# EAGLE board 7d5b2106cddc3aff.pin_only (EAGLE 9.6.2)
REV: A

Size 17.78 x 12.7 mm. Coordinates in mm from the lower left corner, seen from the top.
Outline: 0,10.16 0,2.54 arc90 2.54,0 15.24,0 arc90 17.78,2.54 17.78,10.16 arc90 15.24,12.7 2.54,12.7 arc90 0,10.16
Copper layers (1*16): Top 0.035mm / dielectric 1.5mm / Bottom 0.035mm
Design rules "adafruit *": minimum track width 8mil, minimum drill 15.5mil, track to track 8mil, track to pad 8mil, pad to pad 8mil, via to via 8mil, smd to smd 8mil, copper to edge 10mil, drill to drill 8mil, minimum pad ring 10mil, minimum via ring 8mil, stop-mask expansion 2mil, vias tented up to drill 20mil, thermal gap 10mil
Net classes: 1 highpower: width 0.305 mm, drill 0.483 mm; 2 lowpower: width 0.254 mm, drill 0.483 mm

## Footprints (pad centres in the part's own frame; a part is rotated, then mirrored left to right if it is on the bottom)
0805-NO = smd 1.24 x 1.5: 1 -0.95,0; 2 0.95,0
JST_SH4 = smd 0.6 x 1.55: 1 -1.5,2.006; 2 -0.5,2.006; 3 0.5,2.006; 4 1.5,2.006 | smd 1.2 x 1.8: MT1 -2.8,-1.894; MT2 2.8,-1.894
CHIPLED_0603_NOOUTLINE = smd 0.8 x 0.8: A 0,-0.75; C 0,0.75
FIDUCIAL_1MM = smd 1 x 1: 1 0,0
1X04_ROUND_76 = drill 1 pad 1.93: 1 -3.81,0; 2 -1.27,0; 3 1.27,0; 4 3.81,0
0603-NO = smd 1.075 x 1: 1 -0.85,0; 2 0.85,0
SOLDERJUMPER_CLOSEDWIRE = smd 1.168 x 1.6: 1 -0.762,0; 2 0.762,0 | smd 0.635 x 0.203: WIRE 0,0
SOLDERJUMPER_2WAY_OPEN_NOPASTE = smd 1.168 x 1.6: 1 -1.397,0; 2 0,0; 3 1.397,0
MOUNTINGHOLE_2.5_PLATED = drill 2.5 pad 3.2: P$1 0,0

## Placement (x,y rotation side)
C1  10uF  [0805-NO]  4.7,6.48 90 top
CONN5  STEMMA_I2C_QT  [JST_SH4]  8.89,9.65 180 top
D1  GREEN  [CHIPLED_0603_NOOUTLINE]  2.03,6.6 90 top
FID3  FIDUCIAL_1MM  [FIDUCIAL_1MM]  8.89,10.92 0 top
FID4  FIDUCIAL_1MM  [FIDUCIAL_1MM]  2.29,1.78 0 top
JP1  [1X04_ROUND_76]  8.89,2.54 0 top
PLABEL0  [PLABEL0]  5.08,4.19 0 top
PLABEL1  [PLABEL1]  7.62,0.89 0 top
PLABEL2  [PLABEL2]  10.16,4.19 0 top
PLABEL3  [PLABEL3]  12.7,0.89 0 top
PLABEL4  [PLABEL4]  1.4,7.24 0 top
PLABEL5  [PLABEL5]  3.43,7.49 0 bottom
PLABEL6  [PLABEL6]  16.64,5.46 90 bottom
R1  22K  [0603-NO]  2.16,5.08 0 top
R2  10K  [0603-NO]  13.46,6.86 180 top
R3  10K  [0603-NO]  13.46,5.08 180 top
SJ1  [SOLDERJUMPER_CLOSEDWIRE]  3.56,5.71 180 bottom
SJ2  [SOLDERJUMPER_2WAY_OPEN_NOPASTE]  14.48,5.59 270 bottom
U$1  MOUNTINGHOLE2.5  [MOUNTINGHOLE_2.5_PLATED]  2.54,10.16 0 top
U$2  [ADAFRUIT_3.5MM]  10.92,5.71 0 bottom
U$17  MOUNTINGHOLE2.5  [MOUNTINGHOLE_2.5_PLATED]  15.11,10.03 0 top
U$25  [PCBFEAT-REV-040]  2.41,1.91 0 bottom
U$31  [STEMMAQT]  13.34,9.78 0 bottom

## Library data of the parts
C1 JP1 R1-R3 SJ1 SJ2 U$2 U$25 = microbuilder
CONN5 = adafruit_electromech; LCSC: C2845363
D1 = microbuilder; JLC_ROTATION: 270
FID3 FID4 U$1 U$17 = microbuilder; BOM: EXCLUDE
PLABEL0 PLABEL1-PLABEL6 = pinguin
U$31 = silks

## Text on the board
Pinguin_tBackup: on | VIN | SCL | GND | SDA
Pinguin_bBackup: LED | Pullups

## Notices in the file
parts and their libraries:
microbuilder: This work is placed in the public domain, and may be freely used for commercial and non-commercial work with the following conditions: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
